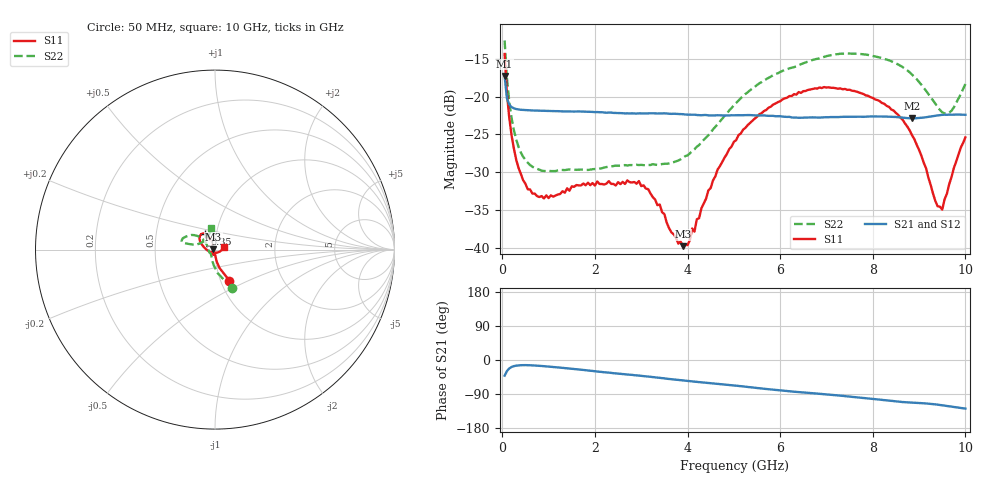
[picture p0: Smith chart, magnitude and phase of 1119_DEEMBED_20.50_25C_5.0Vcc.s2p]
!Hittite Microwave Corp.
!Digital Attenuator/PhaseShifter Rev 1.4.0
!Filename: C:\DATA\DATA\1119_DEEMBED_20.50_25C_5.0Vcc.s2p
!VNA ID: Agilent Technologies,N5224A,MY51441122,A.10.45.03
!Device type:
!2 Port Calibration.
!Temp(C): 25
!Lot Number:
!Serial Number:
!Operator:
!Misc:
!Attenuator:  20.500
# GHZ S DB R 50.0
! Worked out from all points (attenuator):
!   200 points, 50 MHz to 10 GHz, reference 50 ohm
!   highest |S21| = -17.29 dB at 50 MHz (marker M1); lowest = -22.9 dB at 8.85 GHz (marker M2)
!   lowest |S11| = -39.7 dB at 3.9 GHz (marker M3), VSWR 1.02, Z = 49 + j0.128 ohm
!   |S11| at or under -10 dB: start of sweep to end of sweep
!   |S22| runs from -29.8 to -12.6 dB; largest |S21 - S12| = 0.00027
!   S11 on the Smith chart (normalised r, x): 50 MHz: 1.10, -0.40; 6.35 GHz: 0.88, +0.15; 10 GHz: 1.11, +0.04
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0.05  -14.38 -65.1  -17.29 -41.3  -17.30 -41.4  -12.59 -66.4
0.1  -19.58 -76.3  -20.22 -29.4  -20.22 -29.3  -17.55 -83.3
0.2  -25.11 -83.2  -21.38 -18.4  -21.39 -18.4  -22.84 -100.0
0.35  -29.39 -86.3  -21.70 -14.2  -21.70 -14.2  -26.62 -114.0
0.55  -32.24 -90.2  -21.81 -13.7  -21.81 -13.7  -28.72 -125.6
1  -33.40 -98.8  -21.89 -17.3  -21.90 -17.3  -29.79 -136.1
1.75  -31.47 -111.8  -21.98 -26.3  -21.98 -26.3  -29.65 -139.5
2.95  -31.15 -114.3  -22.21 -41.1  -22.22 -41.1  -29.03 -158.5
3.4  -34.24 -129.3  -22.22 -47.1  -22.23 -47.1  -28.96 -171.8
3.9  -39.74 172.7  -22.32 -54.0  -22.33 -54.0  -28.08 168.5
4.15  -37.82 135.5  -22.39 -57.2  -22.40 -57.2  -26.95 157.6
4.65  -29.61 113.0  -22.46 -62.9  -22.48 -63.0  -23.65 143.2
5.05  -25.74 112.6  -22.46 -67.7  -22.48 -67.7  -20.84 139.7
5.55  -22.32 116.0  -22.50 -74.4  -22.51 -74.5  -18.25 142.0
6.35  -19.74 123.1  -22.77 -84.1  -22.78 -84.2  -16.00 149.9
6.7  -19.00 128.6  -22.74 -87.5  -22.75 -87.5  -15.17 154.6
8.35  -21.35 155.5  -22.66 -107.2  -22.66 -107.2  -15.21 168.0
8.85  -25.13 172.3  -22.87 -112.5  -22.87 -112.5  -17.11 167.6
9.35  -33.76 -120.3  -22.53 -117.0  -22.55 -117.1  -20.93 156.9
9.5  -34.91 -70.2  -22.41 -119.5  -22.43 -119.5  -22.07 144.1
9.7  -30.63 -21.0  -22.39 -122.9  -22.40 -122.9  -21.87 121.0
10  -25.38 17.4  -22.40 -128.3  -22.40 -128.2  -18.34 99.5
